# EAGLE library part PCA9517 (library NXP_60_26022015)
Level translating I2C-bus repeater The PCA9517 is a CMOS integrated circuit that provides level shifting between low voltage (down to 0.9 V) and higher voltage (2.7 V to 5.5 V) I2C-bus or SMBus applications. While retaining all the operating modes and features of the I2C-bus system during the level shifts, it also permits extension of the I2C-bus by providing bidirectional buffering for both the data (SDA) and the clock (SCL) lines, thus enabling two buses of 400 pF. Using the PCA9517 enables the system designer to isolate two halves of a bus for both voltage and capacitance. The SDA and SCL pins are over voltage tolerant and are high-impedance when the PCA9517 is unpowered. The 2.7 V to 5.5 V bus B-side drivers behave much like the drivers on the PCA9515A device, while the adjustable voltage bus A-side drivers drive more current and eliminate the static offset voltage. This results in a LOW on the B-side translating into a nearly 0 V LOW on the A-side which accommodates smaller voltage swings of lower voltage logic. The static offset design of the B-side PCA9517 I/O drivers prevent them from being connected to another device that has rise time accelerator including the PCA9510, PCA9511, PCA9512, PCA9513, PCA9514, PCA9515A, PCA9516A, PCA9517 (B-side), or PCA9518. The A-side of two or more PCA9517s can be connected together, however, to allow a star topography with the A-side on the common bus, and the A-side can be connected directly to any other buffer with static or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
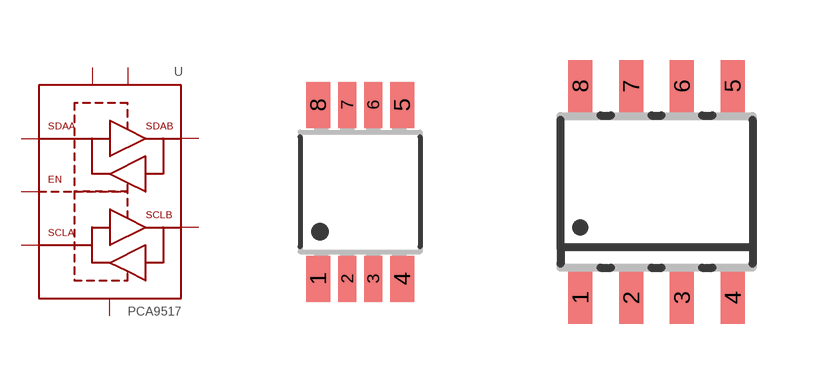
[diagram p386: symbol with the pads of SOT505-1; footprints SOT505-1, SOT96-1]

Designator prefix U

## PCA9517DP  [SOT505-1]
1  VCC(A)  pwr
2  SCLA
3  SDAA
4  GND  pwr
5  EN  in
6  SDAB
7  SCLB
8  VCC(B)  pwr

## PCA9517D  [SOT96-1]
Pads as for SOT505-1

## Footprint SOT505-1 (pad centres in mm)
SOT505-1 TSSOP8: plastic thin shrink small outline package; 8 leads; body width 3 mm JEDEC: -- IEC: --
smd 0.6 x 1.15: 1 -1.05,-2.175; 4 1.05,-2.175; 5 1.05,2.175; 8 -1.05,2.175
smd 0.45 x 1.15: 2 -0.325,-2.175; 3 0.325,-2.175; 6 0.325,2.175; 7 -0.325,2.175

## Footprint SOT96-1 (pad centres in mm)
SOT96-1 SO8: plastic small outline package; 8 leads; body width 3.9 mm JEDEC: MS-012 IEC: 076E03
smd 0.6 x 1.3: 1 -1.905,-2.65; 2 -0.635,-2.65; 3 0.635,-2.65; 4 1.905,-2.65; 5 1.905,2.65; 6 0.635,2.65; 7 -0.635,2.65; 8 -1.905,2.65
